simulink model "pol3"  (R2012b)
settings: Solver=ode45  StartTime=0.0  StopTime=10.0  RelTol=1e-3
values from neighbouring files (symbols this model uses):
  k1 = 100    [aktiv_tilger_1.m]    (also in aktiv_tilger_12.m; aktiv_tilger_2.m = 5; aktiv_tilger_3.m; aktiv_tilger_31.m)
  k2 = 10    [aktiv_tilger_1.m]    (also in aktiv_tilger_12.m; aktiv_tilger_2.m = 10,      c2 = 10; aktiv_tilger_3.m; aktiv_tilger_31.m)
  ki = -Kn(n+1)    [beobachter_2.m]    (also in beobachter_22.m; kalman_12.m = -Kn(3); kalman_13.m = -Kn(4); kalman_d1.m = -Kn(4))
  T1 = 1    [PID_windup1.m]    (also in pol_1.m = -5; pol_2.m = -5; pol_3.m = -5; sprung.m = x(2))
  T2 = 5    [PID_windup1.m]    (also in pol_1.m = 10; pol_2.m = 10; pol_3.m = 10; sprung.m = x(3))

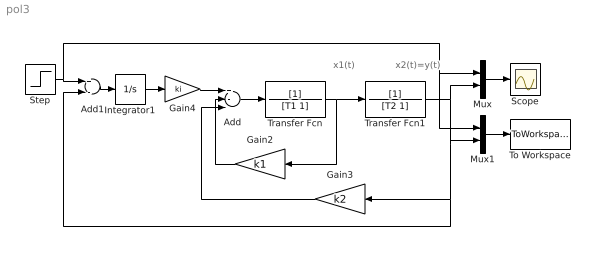
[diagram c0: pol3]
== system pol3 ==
  note: x2(t)=y(t)
  note: x1(t)
  Add : Sum  Inputs=+--
  Add1 : Sum  Inputs=+-
  Gain2 : Gain  Gain=k1
  Gain3 : Gain  Gain=k2
  Gain4 : Gain  Gain=ki
  Integrator1 : Integrator
  Mux : Mux  Inputs=2
  Mux1 : Mux  Inputs=2
  Scope : Scope
  Step : Step  SampleTime=0
  To Workspace : ToWorkspace  VariableName=y  SampleTime=-1  SaveFormat=Structure With Time
  Transfer Fcn : TransferFcn  Denominator=[T1 1]
  Transfer Fcn1 : TransferFcn  Denominator=[T2 1]
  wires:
  Add/1 -> Transfer Fcn/1
  Transfer Fcn/1 -> Gain2/1, Transfer Fcn1/1
  Gain2/1 -> Add/2
  Mux/1 -> Scope/1
  Mux1/1 -> To Workspace/1
  Transfer Fcn1/1 -> Mux/2, Gain3/1, Add1/2, Mux1/2
  Gain3/1 -> Add/3
  Step/1 -> Mux1/1, Mux/1, Add1/1
  Add1/1 -> Integrator1/1
  Integrator1/1 -> Gain4/1
  Gain4/1 -> Add/1
